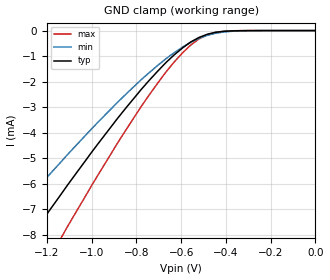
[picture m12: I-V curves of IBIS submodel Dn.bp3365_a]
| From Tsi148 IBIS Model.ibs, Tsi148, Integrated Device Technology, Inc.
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[Submodel]  Dn.bp3365_a
Submodel_type   Dynamic_clamp
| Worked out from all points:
|   GND clamp passes 1 mA (typ) near -0.64 V on its own axis
[GND Clamp]   | Note: Vtable =  Vout
| Voltage   I(typ)   I(min)   I(max)
-3.6V     -39.98mA   -31.93mA   -49.1mA
-1.437V   -10.19mA   -8.115mA   -12.8mA
-1.4V     -9.714mA   -7.742mA   -12.22mA
-1.253V   -7.85mA    -6.272mA   -9.909mA
-1.143V   -6.486mA   -5.199mA   -8.215mA
-1.107V   -6.039mA   -4.847mA   -7.659mA
-777mV    -2.289mA   -1.911mA   -2.952mA
-667mV    -1.244mA   -1.095mA   -1.611mA
-557mV    -446uA     -456uA     -564uA
-483mV    -144uA     -186uA     -164uA
-410mV    -30uA      -55uA      -27uA
0V        0A         0A         0A
